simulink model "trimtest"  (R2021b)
settings: Solver=ode45  StartTime=0.0  StopTime=10  RelTol=1e-3  AbsTol=1e-6
StartFcn:
  | rand; global x_tr
model workspace (MAT data in the model file):
  initial_input_in_model_workspace = [0 0.5 0.5 0.5 0.5 0.5 0.5 0.500000000001 0]
  initial_state_in_model_workspace : object (value not decoded)
undefined symbols (not defined in the file or in its folder): i

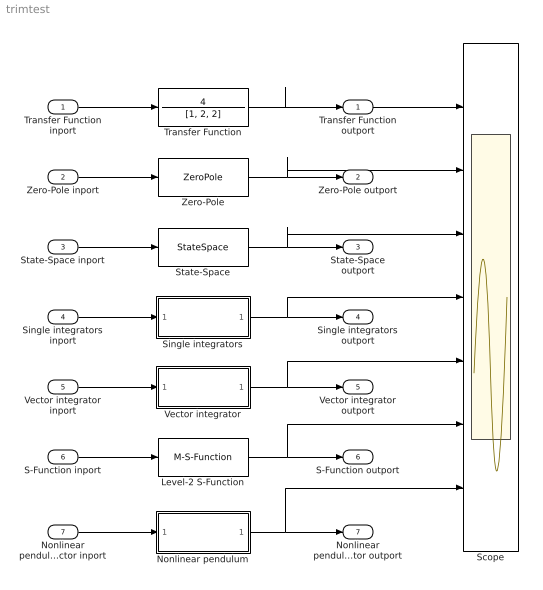
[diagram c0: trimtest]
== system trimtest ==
  Transfer Function inport : Inport
  Zero-Pole inport : Inport  Port=2
  State-Space inport : Inport  Port=3
  Single integrators inport : Inport  Port=4
  Vector integrator inport : Inport  Port=5
  S-Function inport : Inport  Port=6
  Nonlinear pendulum vector inport : Inport  Port=7
  Level-2 S-Function : M-S-Function  FunctionName=second_order_2
  Nonlinear pendulum : Subsystem
  Scope : Scope  NumInputPorts=7
  Single integrators : Subsystem
  State-Space : StateSpace  A=[0, 1; -2, -2]  B=[0; 4]  C=[1, 0]  D=0  InitialCondition=0
  Transfer Function : TransferFcn  Numerator=4  Denominator=[1, 2, 2]
  Vector integrator : Subsystem
  Zero-Pole : ZeroPole  Zeros=[]  Poles=[-1+i; -1-i]  Gain=4
  Transfer Function outport : Outport
  Zero-Pole outport : Outport  Port=2
  State-Space outport : Outport  Port=3
  Single integrators outport : Outport  Port=4
  Vector integrator outport : Outport  Port=5
  S-Function outport : Outport  Port=6
  Nonlinear pendulum vector outport : Outport  Port=7
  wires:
  Vector integrator inport/1 -> Vector integrator/1(In1)
  S-Function inport/1 -> Level-2 S-Function/1
  Single integrators inport/1 -> Single integrators/1(In1)
  Transfer Function inport/1 -> Transfer Function/1
  Zero-Pole inport/1 -> Zero-Pole/1
  State-Space inport/1 -> State-Space/1
  Vector integrator/1(Out1) -> Scope/5, Vector integrator outport/1
  Level-2 S-Function/1 -> Scope/6, S-Function outport/1
  State-Space/1 -> Scope/3, State-Space outport/1
  Zero-Pole/1 -> Scope/2, Zero-Pole outport/1
  Transfer Function/1 -> Scope/1, Transfer Function outport/1
  Single integrators/1(Out1) -> Scope/4, Single integrators outport/1
  Nonlinear pendulum/1(Out1) -> Scope/7, Nonlinear pendulum vector outport/1
  Nonlinear pendulum vector inport/1 -> Nonlinear pendulum/1(In1)

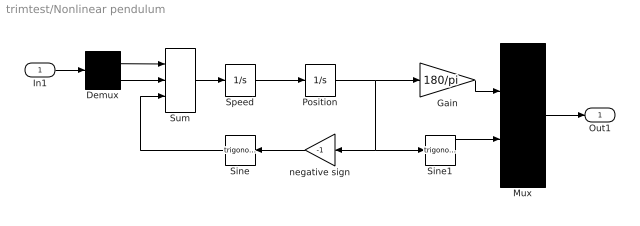
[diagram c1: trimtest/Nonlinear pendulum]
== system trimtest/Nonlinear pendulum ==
  In1 : Inport
  Demux : Demux  Outputs=2
  Gain : Gain  Gain=180/pi  SaturateOnIntegerOverflow=on
  Mux : Mux  Inputs=2
  Position : Integrator
  Sine : Trigonometry
  Sine1 : Trigonometry
  Speed : Integrator
  Sum : Sum  Inputs=3  InputSameDT=on  SaturateOnIntegerOverflow=on
  negative sign : Gain  Gain=-1  SaturateOnIntegerOverflow=on
  Out1 : Outport  InitialOutput=0
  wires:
  Demux/2 -> Sum/2
  Sine/1 -> Sum/3
  Position/1 -> Gain/1, negative sign/1, Sine1/1
  Demux/1 -> Sum/1
  Sum/1 -> Speed/1
  Gain/1 -> Mux/1
  Sine1/1 -> Mux/2
  Speed/1 -> Position/1
  negative sign/1 -> Sine/1
  Mux/1 -> Out1/1
  In1/1 -> Demux/1

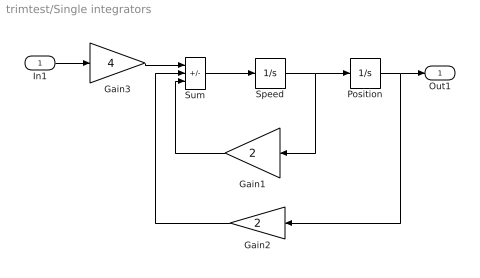
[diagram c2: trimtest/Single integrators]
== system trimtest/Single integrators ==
  In1 : Inport
  Gain1 : Gain  Gain=2  SaturateOnIntegerOverflow=on
  Gain2 : Gain  Gain=2  SaturateOnIntegerOverflow=on
  Gain3 : Gain  Gain=4  SaturateOnIntegerOverflow=on
  Position : Integrator
  Speed : Integrator
  Sum : Sum  Inputs=+--  InputSameDT=on  SaturateOnIntegerOverflow=on
  Out1 : Outport  InitialOutput=0
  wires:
  In1/1 -> Gain3/1
  Sum/1 -> Speed/1
  Gain1/1 -> Sum/3
  Speed/1 -> Position/1, Gain1/1
  Gain2/1 -> Sum/2
  Position/1 -> Gain2/1, Out1/1
  Gain3/1 -> Sum/1

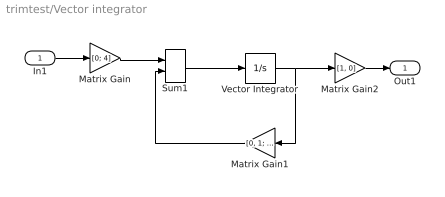
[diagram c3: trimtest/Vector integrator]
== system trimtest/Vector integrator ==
  In1 : Inport
  Matrix Gain : Gain  Gain=[0; 4]  Multiplication=Matrix(K*u)  SaturateOnIntegerOverflow=on
  Matrix Gain1 : Gain  Gain=[0, 1; -2, -2]  Multiplication=Matrix(K*u)  SaturateOnIntegerOverflow=on
  Matrix Gain2 : Gain  Gain=[1, 0]  Multiplication=Matrix(K*u)  SaturateOnIntegerOverflow=on
  Sum1 : Sum  InputSameDT=on  SaturateOnIntegerOverflow=on
  Vector Integrator : Integrator  InitialCondition=[0 0]
  Out1 : Outport  InitialOutput=0
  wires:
  In1/1 -> Matrix Gain/1
  Sum1/1 -> Vector Integrator/1
  Matrix Gain/1 -> Sum1/1
  Vector Integrator/1 -> Matrix Gain2/1, Matrix Gain1/1
  Matrix Gain1/1 -> Sum1/2
  Matrix Gain2/1 -> Out1/1
